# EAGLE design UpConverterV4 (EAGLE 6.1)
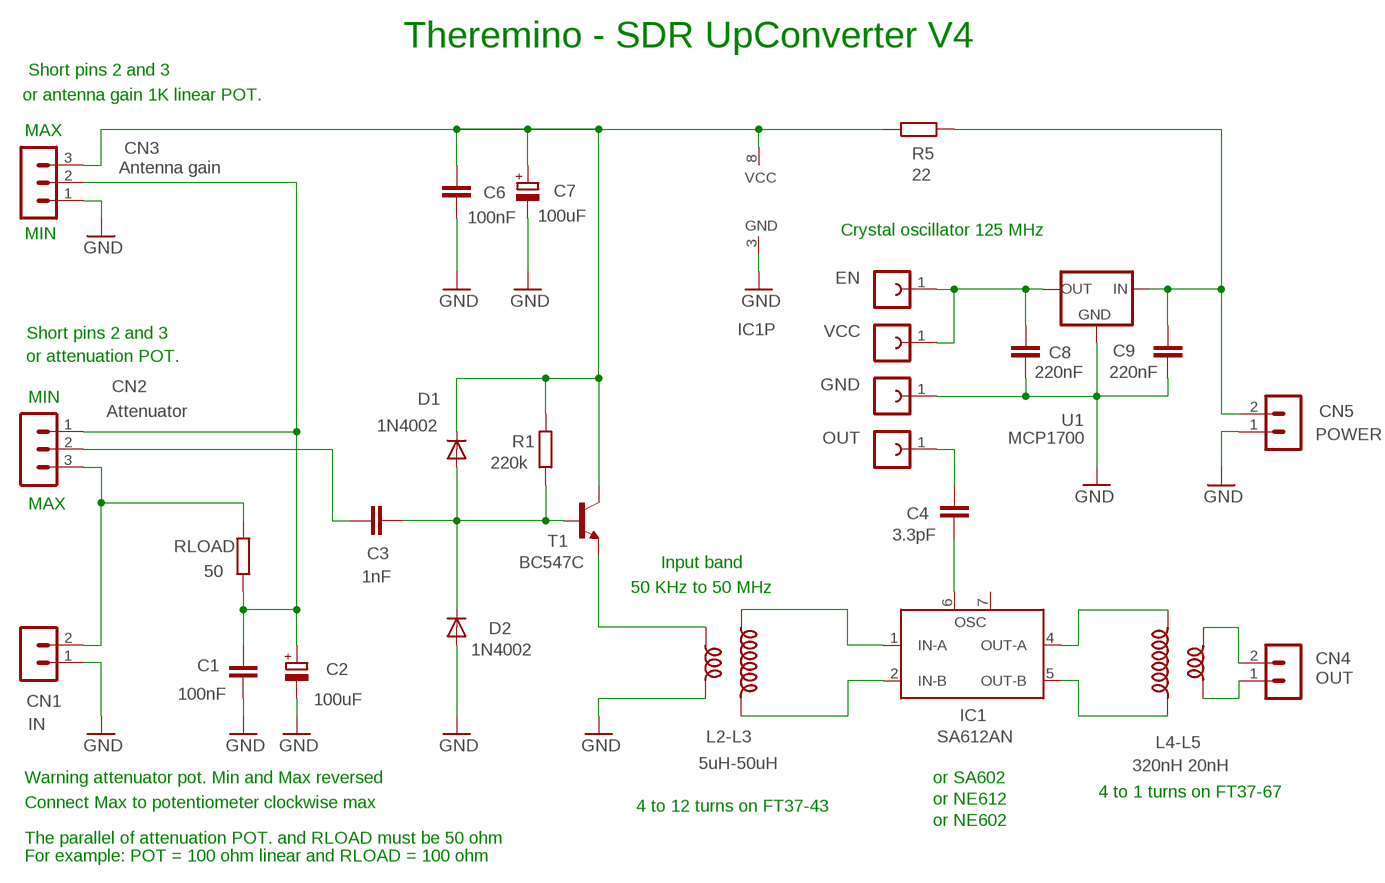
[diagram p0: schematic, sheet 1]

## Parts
C1  100nF  C-EU050-024X044  [C050-024X044]
C2  100uF  CPOL-EUE2-5B  [E2-5B]
C3  1nF  C-EU050-024X044  [C050-024X044]
C4  3.3pF  C-EU050-024X044  [C050-024X044]
C6  100nF  C-EU050-024X044  [C050-024X044]
C7  100uF  CPOL-EUE2-5B  [E2-5B]
C8  220nF  C-EU050-024X044  [C050-024X044]
C9  220nF  C-EU050-024X044  [C050-024X044]
CN1  IN  MA02-1L2  [MA02-1_L2]
CN2  Attenuator  MA03-1L3  [MA03-1_L3]
CN3  Antenna gain  MA03-1L3  [MA03-1_L3]
CN4  OUT  MA02-1N  [MA02-1]
CN5  POWER  MA02-1N  [MA02-1]
D1  1N4002  DIODE-DO34-7  [DO34-7]
D2  1N4002  DIODE-DO34-7  [DO34-7]
IC1  SA612AN  [DIL08]
L2-L3  5uH-50uH  INDUCTOR_DUALTOR2_REV2  [TOROID_2]
L4-L5  320nH 20nH  INDUCTOR_DUALTOR2_REV1  [TOROID_2]
QZ1  EN  FE01-1  [FE01-1]
QZ2  GND  FE01-1  [FE01-1]
QZ3  OUT  FE01-1  [FE01-1]
QZ4  VCC  FE01-1  [FE01-1]
R1  220k  R-EU_0204/7  [0204/7]
R5  22  R-EU_0204/7  [0204/7]
RLOAD  50  R-EU_0204/7  [0204/7]
T1  BC547C  -NPN-TO92-CBE  [TO92-CBE]
U1  MCP1700  MCP1700L1  [TO92L1]

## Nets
GND: C1.2 C2.- C6.2 C7.- C8.2 C9.2 CN1.1 CN3.1 CN5.1 D2.A IC1.3(GND) L2-L3.3 QZ2.1 U1.3(GND)
L4-L5: IC1.5(OUT-B) L4-L5.1
N$1: C9.1 CN5.2 R5.2 U1.2(IN)
N$2: CN1.2 CN2.3 RLOAD.1
N$3: C3.2 D1.A D2.C R1.1 T1.B
N$4: IC1.2(IN-B) L2-L3.2
N$5: C6.1 C7.+ CN3.3 D1.C IC1.8(VCC) R1.2 R5.1 T1.C
N$6: L2-L3.4 T1.E
N$7: C1.1 C2.+ CN2.1 CN3.2 RLOAD.2
N$8: IC1.1(IN-A) L2-L3.1
N$9: C4.1 IC1.6(OSC)
N$10: C4.2 QZ3.1
N$11: IC1.4(OUT-A) L4-L5.2
N$12: CN4.1 L4-L5.4
N$13: CN4.2 L4-L5.3
N$14: C3.1 CN2.2
N$17: C8.1 QZ1.1 QZ4.1 U1.1(OUT)
Unconnected: IC1.7(OSC')

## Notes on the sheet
- Theremino - SDR UpConverter V4
- Short pins 2 and 3
- or antenna gain 1K linear POT.
- MAX
- MIN | Crystal oscillator 125 MHz
- Short pins 2 and 3
- or attenuation POT.
- MIN
- MAX
- Input band
- 50 KHz to 50 MHz
- Warning attenuator pot. Min and Max reversed | or SA602
- 4 to 1 turns on FT37-67
- Connect Max to potentiometer clockwise max | or NE612
- 4 to 12 turns on FT37-43
- or NE602
- The parallel of attenuation POT. and RLOAD must be 50 ohm
- For example: POT = 100 ohm linear and RLOAD = 100 ohm

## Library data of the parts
C1 C3 C4 C6 C8 C9 = 00-LIVIO:C-EU: CAPACITOR, European symbol
C2 C7 = 00-LIVIO:CPOL-EU: POLARIZED CAPACITOR, European symbol
CN1 CN4 CN5 = 03-con-lstb-M:MA02-1: PIN HEADER
CN2 CN3 = 03-con-lstb-M:MA03-1: PIN HEADER
D1 D2 = 00-LIVIO:DIODE-: DIODE
IC1 = linear:SA612A: Double-balanced mixer and oscillator NE612/SA612 Source: www-eu2.semiconductors.philips.com/acrobat/datasheets/SA612A.pdf
L2-L3 L4-L5 = 00-LIVIO:INDUCTOR_DUAL
QZ1-QZ4 = 02-con-lsta-F:FE01-1: FEMALE HEADER
R1 R5 RLOAD = 00-LIVIO:R-EU_: RESISTOR, European symbol
T1 = 00-LIVIO:*-NPN-: NPN Transistror
U1 = 00-LIVIO:MCP1700: Linear regulator Quescient courrent 1.8uA Input 2.3v to 6v Output 1.2v 1.8v 2.5v 3.0v 3.3v 5.0v

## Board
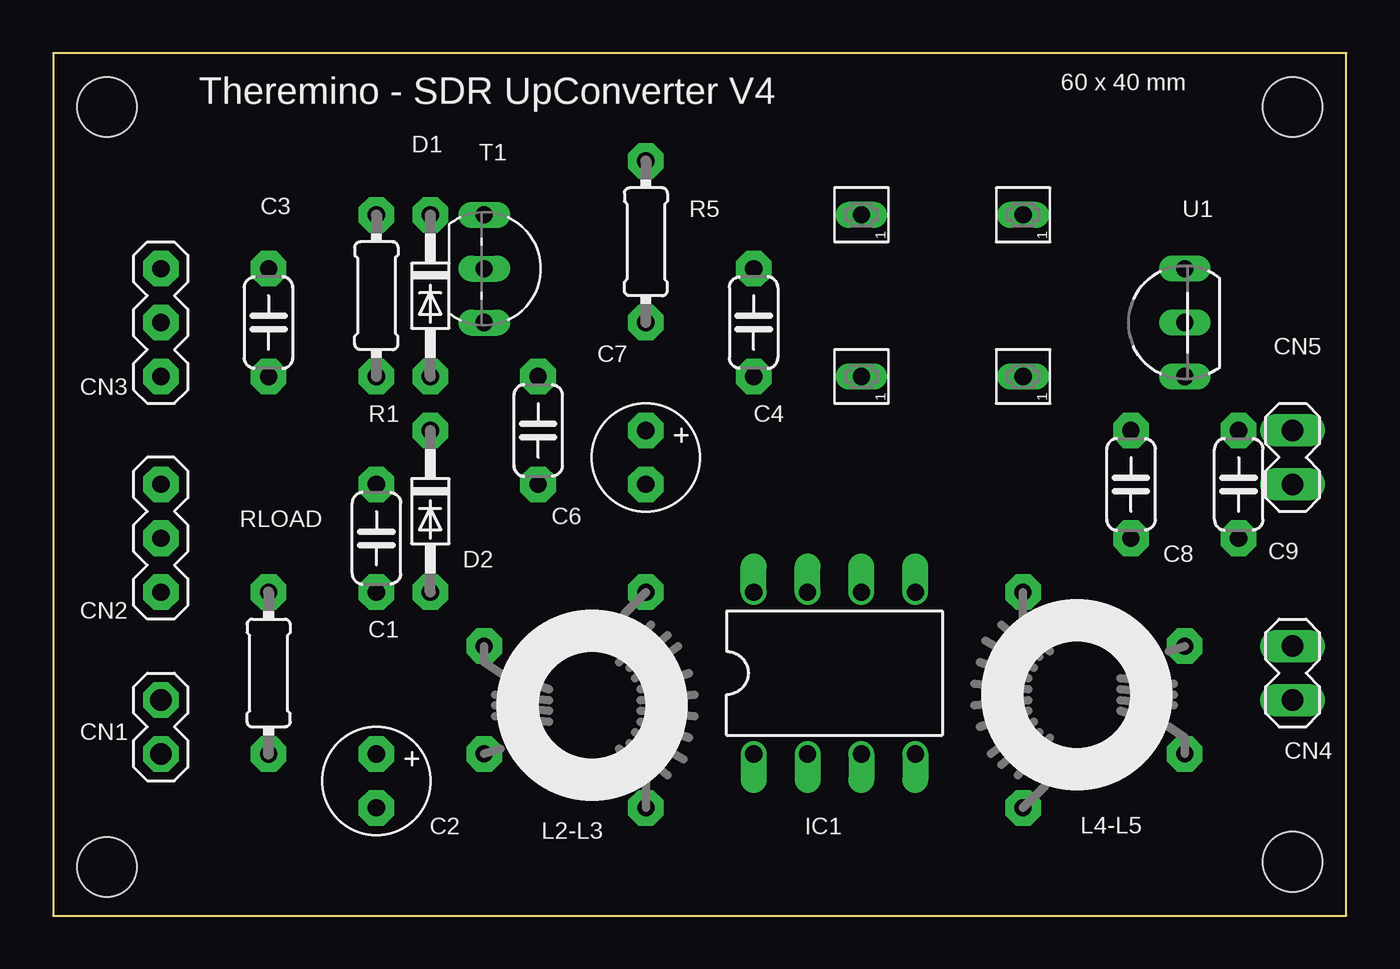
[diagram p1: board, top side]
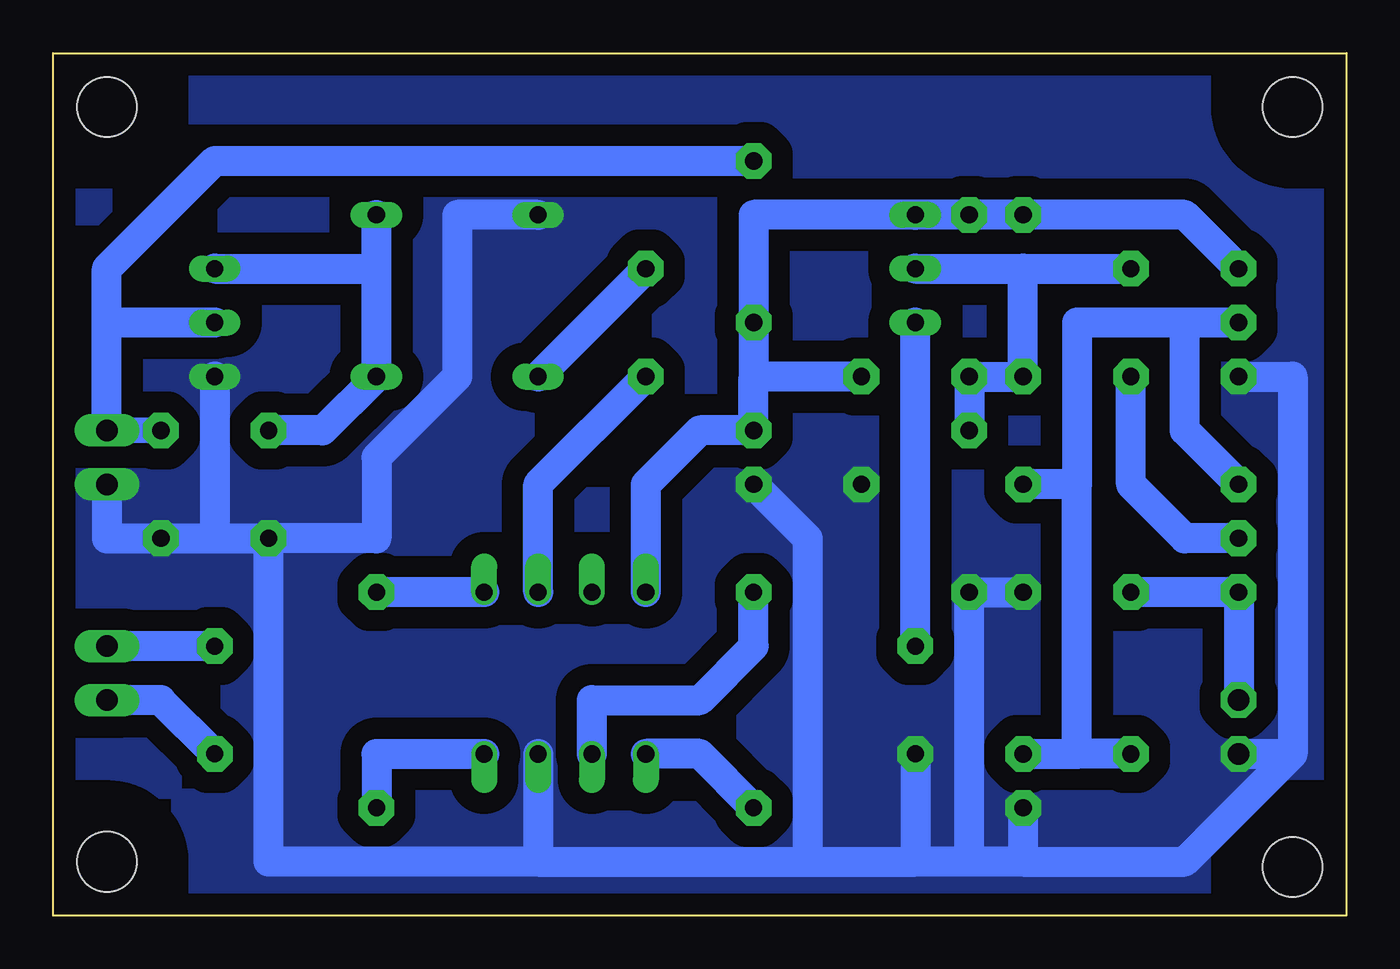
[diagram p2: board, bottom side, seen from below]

Size 60.96 x 40.64 mm. Coordinates in mm from the lower left corner, seen from the top.
Outline: 0,0 60.96,0 60.96,40.64 0,40.64 0,0
Copper layers (1*16): Top 0.035mm / dielectric 1.5mm / Bottom 0.035mm
Design rules: minimum track width 10mil, minimum drill 0.6mm, track to track 8mil, track to pad 8mil, pad to pad 8mil, via to via 8mil, smd to smd 8mil, copper to edge 31mil, drill to drill 8mil, minimum pad ring 5mil, minimum via ring 8mil, stop-mask expansion 4mil, vias tented up to drill 0mil, thermal gap 47mil
Holes 2.8 mm at 2.54,38.1 58.42,38.1 58.42,2.54 2.54,2.29
bRestrict: 12 lines

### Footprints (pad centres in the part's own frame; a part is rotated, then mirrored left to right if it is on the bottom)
C050-024X044 = drill 0.813 pad 1.676 octagon: 1 -2.54,0; 2 2.54,0
E2-5B = drill 0.813 pad 1.676 octagon: + -1.27,0; - 1.27,0
MA02-1_L2 = drill 1.016 pad 1.676 octagon: 1 -1.27,0; 2 1.27,0
MA03-1_L3 = drill 0.813 pad 1.676 octagon: 1 -2.54,0; 2 0,0; 3 2.54,0
MA02-1 = drill 1.016 long: 1 -1.27,0; 2 1.27,0
DO34-7 = drill 0.813 pad 1.676 octagon: A 3.81,0; C -3.81,0
DIL08 = drill 0.813 offset: 1 -3.81,-3.81; 2 -1.27,-3.81; 3 1.27,-3.81; 4 3.81,-3.81; 5 3.81,3.81; 6 1.27,3.81; 7 -1.27,3.81; 8 -3.81,3.81
TOROID_2 = drill 0.8 pad 1.676 octagon: 1 -2.54,5.08; 2 -2.54,-5.08; 3 5.08,2.54; 4 5.08,-2.54
FE01-1 = drill 0.813 long: 1 0,0
0204/7 = drill 0.813 pad 1.676 octagon: 1 -3.81,0; 2 3.81,0
TO92-CBE = drill 0.813 long: B 0,0; C -2.54,0; E 2.54,0
TO92L1 = drill 0.813 long: 1 2.54,0; 2 0,0; 3 -2.54,0

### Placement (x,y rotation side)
C1  15.24,17.78 270 top
C2  15.24,6.35 270 top
C3  10.16,27.94 90 top
C4  33.02,27.94 90 top
C6  22.86,22.86 270 top
C7  27.94,21.59 270 top
C8  50.8,20.32 270 top
C9  55.88,20.32 270 top
CN1  5.08,8.89 90 top
CN2  5.08,17.78 270 top
CN3  5.08,27.94 90 top
CN4  58.42,11.43 90 top
CN5  58.42,21.59 90 top
D1  17.78,29.21 270 top
D2  17.78,19.05 270 top
IC1  36.83,11.43 0 top
L2-L3  25.4,10.16 180 top
L4-L5  48.26,10.16 0 top
QZ1  45.72,33.02 90 top
QZ2  38.1,33.02 90 top
QZ3  38.1,25.4 90 top
QZ4  45.72,25.4 90 top
R1  15.24,29.21 90 top
R5  27.94,31.75 90 top
RLOAD  10.16,11.43 270 top
T1  20.32,30.48 270 top
U1  53.34,27.94 90 top

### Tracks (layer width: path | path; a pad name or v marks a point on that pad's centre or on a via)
GND
  Bottom 1.422: 15.24,2.54 7.62,2.54 2.54,7.62 | IC1.3 38.1,2.54 | 38.1,2.54 25.4,2.54 | 25.4,2.54 20.32,2.54 | 38.1,2.54 50.8,2.54 C8.2 | L2-L3.3 20.32,2.54 | QZ2.1 41.91,33.02 41.91,25.4 45.72,21.59 45.72,17.78 C8.2 | CN5.1 58.42,17.78 C9.2 53.34,17.78 | 53.34,17.78 C8.2 | U1.3 53.34,17.78 | 17.78,2.54 20.32,2.54 | CN3.1 2.54,25.4 2.54,7.62 | CN1.1 2.54,7.62 | C2.- 15.24,2.54 | 25.4,2.54 25.4,17.78 C7.- | 15.24,2.54 17.78,2.54 | 17.78,2.54 D2.A C1.2
  pour Bottom (isolate 1, rank 6, no thermals): -1,-1 61.96,-1 61.96,41.64 -1,41.64
L4-L5
  Bottom 1.422: 43.18,15.24 IC1.5 L4-L5.1
N$1
  Bottom 1.2: CN5.2 C9.1
  Bottom 1.422: R5.2 53.34,35.56 58.42,30.48 58.42,27.94 | CN5.2 58.42,27.94 | U1.2 58.42,27.94
N$2
  Bottom 1.422: RLOAD.1 CN2.3 CN1.2
N$3
  Bottom 1.422: T1.B 15.24,30.48 | 15.24,30.48 R1.1 D1.A D2.C | 15.24,30.48 C3.2
N$4
  Bottom 1.422: IC1.2 35.56,10.16 30.48,10.16 27.94,12.7 L2-L3.2
N$5
  Bottom 1.422: IC1.8 33.02,20.32 30.48,22.86 C7.+ 27.94,25.4 | 27.94,25.4 R5.1 27.94,33.02 T1.C D1.C | CN3.3 7.62,33.02 D1.C | R1.2 D1.C | C6.1 27.94,25.4
N$6
  Bottom 1.422: L2-L3.4 T1.E
N$7
  Bottom 1.422: RLOAD.2 12.7,7.62 | 12.7,7.62 12.7,20.32 | CN3.2 7.62,27.94 | 7.62,27.94 12.7,27.94 12.7,20.32 | 12.7,20.32 C1.1 | CN2.1 7.62,22.86 7.62,27.94 | C2.+ 12.7,7.62
N$8
  Bottom 1.422: IC1.1 30.48,7.62 L2-L3.1
N$9
  Bottom 1.422: IC1.6 38.1,20.32 C4.1
N$10
  Bottom 1.422: C4.2 QZ3.1
N$11
  Bottom 1.422: L4-L5.2 45.72,7.62 IC1.4
N$12
  Bottom 1.422: L4-L5.4 55.88,10.16 CN4.1
N$13
  Bottom 1.422: L4-L5.3 CN4.2
N$14
  Bottom 1.422: CN2.2 7.62,17.78 10.16,20.32 C3.1
N$17
  Bottom 1.422: 45.72,30.48 QZ4.1 48.26,22.86 C8.1 | 45.72,30.48 QZ1.1 | U1.1 45.72,30.48

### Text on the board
tNames: 60 x 40 mm | Theremino - SDR UpConverter V4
